FUNCTION_BLOCK PROCESS
VAR_INPUT
	ENABLE:BOOL;
	NEXTSTEP_EN:BOOL;
	Alarm_RST:BOOL;
	PMStableTime:INT;
	STEP_DATA:RecipeEachStep;
END_VAR
VAR_OUTPUT
	
	//APC
	APC_PRESSURE:REAL;
	APC_POSITION:REAL;
	APC_CONTROL_MODE:SINT;
	
	//MFC
	MFC1_SV:REAL;
	MFC2_SV:REAL;
	MFC3_SV:REAL;
	MFC4_SV:REAL;
	MFC5_SV:REAL;
	MFC6_SV:REAL;
	MFC7_SV:REAL;
	MFC8_SV:REAL;	
	MFC9_SV:REAL;	
	
	//HEATER
	WALL_TEMP:REAL;
	LID_TEMP:REAL;
	STAGE_TEMP1,
	STAGE_TEMP2,
	STAGE_TEMP3,
	STAGE_TEMP4:REAL;
	
	//STEP
	STEP_TIME_OUT:BOOL;
	STEP_ERR:BOOL;
	NEXTSTEP:BOOL;
	
	//Tolerance
	PRESSURE_WARNING:BOOL;
	PRESSURE_ALARM:BOOL;
	
	MFC1_WARNING:BOOL;
	MFC1_Alarm:BOOL;
	
	MFC2_WARNING:BOOL;
	MFC2_Alarm:BOOL;
	
	MFC3_WARNING:BOOL;
	MFC3_Alarm:BOOL;
	
	MFC4_WARNING:BOOL;
	MFC4_Alarm:BOOL;
	
	MFC5_WARNING:BOOL;
	MFC5_Alarm:BOOL;
	
	MFC6_WARNING:BOOL;
	MFC6_Alarm:BOOL;
	
	MFC7_WARNING:BOOL;
	MFC7_Alarm:BOOL;
	
	MFC8_WARNING:BOOL;
	MFC8_Alarm:BOOL;
	
	MFC9_WARNING:BOOL;
	MFC9_Alarm:BOOL;
	
	WALL_TEMP_WARNING:BOOL;
	WALL_TEMP_Alarm:BOOL;
		
	LID_TEMP_WARNING:BOOL;
	LID_TEMP_Alarm:BOOL;
	
	STAGE_TEMP1_WARNING:BOOL;
	STAGE_TEMP1_Alarm:BOOL;
	
	STAGE_TEMP2_WARNING:BOOL;
	STAGE_TEMP2_Alarm:BOOL;
	
	STAGE_TEMP3_WARNING:BOOL;
	STAGE_TEMP3_Alarm:BOOL;
	
	STAGE_TEMP4_WARNING:BOOL;
	STAGE_TEMP4_Alarm:BOOL;
	
END_VAR
VAR
	STEP_TIME:TON;
	STEP_TIME_DONE:BOOL;
	
	COMPLETION:INT;
	
	//Tolerance
	TOL_PRESSURE_PERCENT:Tolerance;
	TOL_PRESSURE_VALUE_EN:BOOL;
	TOL_PRESSURE_PERCENT_EN:BOOL;
	
	TOL_MFC1:Tolerance;
	TOL_MFC2:Tolerance;
	TOL_MFC3:Tolerance;
	//TOL_MFC4:Tolerance;
	TOL_MFC5:Tolerance;
	TOL_MFC6:Tolerance;
	TOL_MFC7:Tolerance;
	//TOL_MFC8:Tolerance;
	//TOL_MFC9:Tolerance;
	TOL_MFC_VALUE_EN:BOOL;
	TOL_MFC_PERCENT_EN:BOOL;

	TOL_WALL_TEMP:Tolerance;

	TOL_LID_TEMP:Tolerance;

	TOL_STAGE_TEMP1:Tolerance;	
	TOL_STAGE_TEMP2:Tolerance;
	TOL_STAGE_TEMP3:Tolerance;	
	TOL_STAGE_TEMP4:Tolerance;
	
	TOL_HEATER_VALUE_EN:BOOL;
	TOL_HEATER_PERCENT_EN:BOOL;
	
	TON_STEP_TIME:TON;
	TON_STEP_TIME_EN:BOOL;
	
	WARNING_OCC:BOOL;
	ALARM_OCC:BOOL;
	
	i:INT;
	
	STABLE_DONE:BOOL;
	EN_TRIG:R_TRIG;
	TON_STABLE_PROCESS:TON;
	
	CHAMBER_TEMP_MIN_VALUE:REAL;
	STAGE_EDGE_TEMP_MIN_VALUE:REAL;
	STAGE_CENTER_TEMP_MIN_VALUE:REAL;
		
END_VAR

//NOT ENABLE
	IF NOT ENABLE 
		THEN
		i:=0;
		STEP_ERR:=FALSE;
		STEP_TIME_OUT:=FALSE;
		NEXTSTEP:=FALSE;
		TON_STEP_TIME_EN:=FALSE;
	END_IF;
	
//初始化
	EN_TRIG(CLK:= ENABLE, Q=> );
	IF EN_TRIG.Q OR NEXTSTEP_EN
		THEN
		i:=1;
		STEP_ERR:=FALSE;
		STEP_TIME_OUT:=FALSE;
		NEXTSTEP:=FALSE;
		TON_STEP_TIME_EN:=TRUE;
	END_IF;

	
//STEP开始时赋值
	IF  ENABLE AND NOT STEP_TIME_DONE
	THEN
	//APC
	IF 		STEP_DATA.LstUnit.Pressure.PressureUnitMode = 'Pressure' 
			THEN
			APC_PRESSURE:=STEP_DATA.LstUnit.Pressure.StartValue;
			APC_CONTROL_MODE:=5;
			ELSIF 	
			STEP_DATA.LstUnit.Pressure.PressureUnitMode = 'Position'	
			THEN
			APC_POSITION:=STEP_DATA.LstUnit.Pressure.StartValue;
			APC_CONTROL_MODE:=2;
	END_IF
	
	IF 		STEP_DATA.LstUnit.Pressure.ToleranceMode = 'Value' 
			THEN
			TOL_PRESSURE_VALUE_EN:=TRUE;
			TOL_PRESSURE_PERCENT_EN:=FALSE;
			ELSIF 	
			STEP_DATA.LstUnit.Pressure.ToleranceMode = 'Percent'	
			THEN
			TOL_PRESSURE_VALUE_EN:=FALSE;
			TOL_PRESSURE_PERCENT_EN:=TRUE;
	END_IF
	
	//MFC
	IF 		STEP_DATA.LstUnit.GAS.ToleranceMode = 'Value' 
			THEN
			TOL_MFC_VALUE_EN:=TRUE;
			TOL_MFC_PERCENT_EN:=FALSE;
			ELSIF 	
			STEP_DATA.LstUnit.GAS.ToleranceMode = 'Percent'	
			THEN
			TOL_MFC_VALUE_EN:=FALSE;
			TOL_MFC_PERCENT_EN:=TRUE;
	END_IF
	
	MFC1_SV:=INT_TO_REAL(STEP_DATA.LstUnit.GAS.Gas1);
	MFC2_SV:=INT_TO_REAL(STEP_DATA.LstUnit.GAS.Gas2);
	MFC3_SV:=INT_TO_REAL(STEP_DATA.LstUnit.GAS.Gas3);
	MFC4_SV:=INT_TO_REAL(STEP_DATA.LstUnit.GAS.Gas4);	
	MFC5_SV:=INT_TO_REAL(STEP_DATA.LstUnit.GAS.Gas5);
	MFC6_SV:=INT_TO_REAL(STEP_DATA.LstUnit.GAS.Gas6);
	MFC7_SV:=INT_TO_REAL(STEP_DATA.LstUnit.GAS.Gas7);
	MFC8_SV:=INT_TO_REAL(STEP_DATA.LstUnit.GAS.Gas8);	
	MFC9_SV:=INT_TO_REAL(STEP_DATA.LstUnit.GAS.Gas9);
	
	//HEATER
	IF 		STEP_DATA.LstUnit.Heater.ToleranceMode = 'Value' 
			THEN
			TOL_HEATER_VALUE_EN:=TRUE;
			TOL_HEATER_PERCENT_EN:=FALSE;
			ELSIF 	
			STEP_DATA.LstUnit.Heater.ToleranceMode = 'Percent'	
			THEN
			TOL_HEATER_VALUE_EN:=FALSE;
			TOL_HEATER_PERCENT_EN:=TRUE;
	END_IF
	
	WALL_TEMP:=INT_TO_REAL(STEP_DATA.LstUnit.Heater.WallTemp);
	LID_TEMP:=INT_TO_REAL(STEP_DATA.LstUnit.Heater.LidTemp);
	STAGE_TEMP1:=INT_TO_REAL(STEP_DATA.LstUnit.Heater.StageTemp1);
	STAGE_TEMP2:=INT_TO_REAL(STEP_DATA.LstUnit.Heater.StageTemp2);
	STAGE_TEMP3:=INT_TO_REAL(STEP_DATA.LstUnit.Heater.StageTemp3);
	STAGE_TEMP4:=INT_TO_REAL(STEP_DATA.LstUnit.Heater.StageTemp4);
	END_IF;
	
// Lifter
	GV.NDO.AV110 :=	STEP_DATA.Lifter_Up AND NOT STEP_DATA.Lifter_Down;
	GV.NDO.AV109 :=	FALSE;
	
//取最小值
		IF 
		GV.AI.Chamber_Temp1<=GV.AI.Chamber_Temp2 AND GV.AI.Chamber_Temp1<=GV.AI.Chamber_Temp3
		THEN 
		CHAMBER_TEMP_MIN_VALUE:=GV.AI.Chamber_Temp1;
		ELSIF 
		GV.AI.Chamber_Temp2<=GV.AI.Chamber_Temp1 AND GV.AI.Chamber_Temp2<=GV.AI.Chamber_Temp3
		THEN
		CHAMBER_TEMP_MIN_VALUE:=GV.AI.Chamber_Temp2;
		ELSIF
		GV.AI.Chamber_Temp3<=GV.AI.Chamber_Temp2 AND GV.AI.Chamber_Temp3<=GV.AI.Chamber_Temp1
		THEN
		CHAMBER_TEMP_MIN_VALUE:=GV.AI.Chamber_Temp3;
	END_IF
	
//Tolerance
	TOL_PRESSURE_PERCENT(
		ENABLE:= TOL_PRESSURE_PERCENT.SV>0	AND ENABLE,
		STEP_TYPE:=	STEP_DATA.Completion,
		STEP_TIME:=	STEP_DATA.StepTime+STEP_DATA.AddTime,
		TOL_V:= TOL_PRESSURE_VALUE_EN, 
		TOL_P:= TOL_PRESSURE_PERCENT_EN, 
		SV:= STEP_DATA.LstUnit.Pressure.StartValue, 
		PV:= GV.AI.	APC.ACTUAL_PRESSURE, 
		WARNING_RANGE:= STEP_DATA.LstUnit.Pressure.StartValueWarningRange, 
		ALARM_RANGE:= STEP_DATA.LstUnit.Pressure.StartValueAlarmRange, 
		DELAY_TIME:=STEP_DATA.LstUnit.Pressure.ToleranceDelayTime,
		RST	:=	Alarm_RST,
		STABLE_TIME := PMStableTime,
		STU_WARNING=> PRESSURE_WARNING, 
		STU_ALARM=> PRESSURE_ALARM, );

	TOL_MFC1(
		ENABLE:= TOL_MFC1.SV>0	AND ENABLE,
		STEP_TYPE:=	STEP_DATA.Completion,
		STEP_TIME:=	STEP_DATA.StepTime+STEP_DATA.AddTime,
		TOL_V:= TOL_MFC_VALUE_EN, 
		TOL_P:= TOL_MFC_PERCENT_EN, 
		SV:= STEP_DATA.LstUnit.GAS.Gas1, 
		PV:= GV.AI.MFC1_Flow, 
		WARNING_RANGE:= STEP_DATA.LstUnit.GAS.Gas1WarningRange, 
		ALARM_RANGE:= STEP_DATA.LstUnit.GAS.Gas1AlarmRange, 
		DELAY_TIME:=STEP_DATA.LstUnit.GAS.ToleranceDelayTime,
		RST	:=	Alarm_RST,
		STABLE_TIME := PMStableTime,
		STU_WARNING=> MFC1_WARNING, 
		STU_ALARM=> MFC1_Alarm, );
(*	
	TOL_MFC2(
		ENABLE:= TOL_MFC2.SV>0	AND ENABLE,
		STEP_TYPE:=	STEP_DATA.Completion,
		STEP_TIME:=	STEP_DATA.StepTime+STEP_DATA.AddTime,
		TOL_V:= TOL_MFC_VALUE_EN, 
		TOL_P:= TOL_MFC_PERCENT_EN, 
		SV:= STEP_DATA.LstUnit.GAS.Gas2, 
		PV:= GV.AI.MFC2_Flow,
		WARNING_RANGE:= STEP_DATA.LstUnit.GAS.Gas2WarningRange, 
		ALARM_RANGE:= STEP_DATA.LstUnit.GAS.Gas2AlarmRange,  
		DELAY_TIME:=STEP_DATA.LstUnit.GAS.ToleranceDelayTime,
		RST	:=	Alarm_RST,
		STABLE_TIME := PMStableTime,
		STU_WARNING=> MFC2_WARNING, 
		STU_ALARM=> MFC2_Alarm, );
	
	TOL_MFC3(
		ENABLE:= TOL_MFC3.SV>0	AND ENABLE,
		STEP_TYPE:=	STEP_DATA.Completion,
		STEP_TIME:=	STEP_DATA.StepTime+STEP_DATA.AddTime,
		TOL_V:= TOL_MFC_VALUE_EN, 
		TOL_P:= TOL_MFC_PERCENT_EN, 
		SV:= STEP_DATA.LstUnit.GAS.Gas3, 
		PV:= GV.AI.MFC3_Flow,
		WARNING_RANGE:= STEP_DATA.LstUnit.GAS.Gas3WarningRange, 
		ALARM_RANGE:= STEP_DATA.LstUnit.GAS.Gas3AlarmRange, 
		DELAY_TIME:=STEP_DATA.LstUnit.GAS.ToleranceDelayTime,
		RST	:=	Alarm_RST,
		STABLE_TIME := PMStableTime,
		STU_WARNING=> MFC3_WARNING, 
		STU_ALARM=> MFC3_Alarm, );
	
	
	TOL_MFC5(
		ENABLE:= TOL_MFC5.SV>0	AND ENABLE,
		STEP_TYPE:=	STEP_DATA.Completion,
		STEP_TIME:=	STEP_DATA.StepTime+STEP_DATA.AddTime,
		TOL_V:= TOL_MFC_VALUE_EN, 
		TOL_P:= TOL_MFC_PERCENT_EN, 
		SV:= STEP_DATA.LstUnit.GAS.Gas5, 
		PV:= GV.AI.MFC5_Flow,
		WARNING_RANGE:= STEP_DATA.LstUnit.GAS.Gas5WarningRange, 
		ALARM_RANGE:= STEP_DATA.LstUnit.GAS.Gas5AlarmRange, 
		DELAY_TIME:=STEP_DATA.LstUnit.GAS.ToleranceDelayTime,
		RST	:=	Alarm_RST, 
		STABLE_TIME := PMStableTime,
		STU_WARNING=> MFC5_WARNING, 
		STU_ALARM=> MFC5_Alarm, );
	
	TOL_MFC6(
		ENABLE:= TOL_MFC6.SV>0	AND ENABLE,
		STEP_TYPE:=	STEP_DATA.Completion,
		STEP_TIME:=	STEP_DATA.StepTime+STEP_DATA.AddTime,
		TOL_V:= TOL_MFC_VALUE_EN, 
		TOL_P:= TOL_MFC_PERCENT_EN, 
		SV:= STEP_DATA.LstUnit.GAS.Gas6, 
		PV:= GV.AI.MFC6_Flow,
		WARNING_RANGE:= STEP_DATA.LstUnit.GAS.Gas6WarningRange, 
		ALARM_RANGE:= STEP_DATA.LstUnit.GAS.Gas6AlarmRange, 
		DELAY_TIME:=STEP_DATA.LstUnit.GAS.ToleranceDelayTime,
		RST	:=	Alarm_RST,
		STABLE_TIME := PMStableTime,
		STU_WARNING=> MFC6_WARNING, 
		STU_ALARM=> MFC6_Alarm, );
	
	TOL_MFC7(
		ENABLE:= TOL_MFC7.SV>0	AND ENABLE,
		STEP_TYPE:=	STEP_DATA.Completion,
		STEP_TIME:=	STEP_DATA.StepTime+STEP_DATA.AddTime,
		TOL_V:= TOL_MFC_VALUE_EN, 
		TOL_P:= TOL_MFC_PERCENT_EN, 
		SV:= STEP_DATA.LstUnit.GAS.Gas7, 
		PV:= GV.AI.MFC7_Flow,
		WARNING_RANGE:= STEP_DATA.LstUnit.GAS.Gas7WarningRange, 
		ALARM_RANGE:= STEP_DATA.LstUnit.GAS.Gas7AlarmRange, 
		DELAY_TIME:=STEP_DATA.LstUnit.GAS.ToleranceDelayTime,
		RST	:=	Alarm_RST,
		STABLE_TIME := PMStableTime,
		STU_WARNING=> MFC7_WARNING, 
		STU_ALARM=> MFC7_Alarm, );
*)
	TOL_WALL_TEMP(
		ENABLE:= ENABLE,
		STEP_TYPE:=	STEP_DATA.Completion,
		STEP_TIME:=	STEP_DATA.StepTime+STEP_DATA.AddTime,
		TOL_V:= TOL_HEATER_VALUE_EN, 
		TOL_P:= TOL_HEATER_PERCENT_EN, 
		SV:= STEP_DATA.LstUnit.Heater.WallTemp, 
		PV:= CHAMBER_TEMP_MIN_VALUE, 
		WARNING_RANGE:= STEP_DATA.LstUnit.Heater.WallTempWaningRange, 
		ALARM_RANGE:= STEP_DATA.LstUnit.Heater.WallTempAlarmRange, 
		DELAY_TIME:=STEP_DATA.LstUnit.Heater.ToleranceDelayTime,
		RST	:=	Alarm_RST,
		STABLE_TIME := PMStableTime,
		STU_WARNING=> WALL_TEMP_WARNING, 
		STU_ALARM=> WALL_TEMP_Alarm, );
	
	TOL_LID_TEMP(
		ENABLE:= ENABLE,
		STEP_TYPE:=	STEP_DATA.Completion,
		STEP_TIME:=	STEP_DATA.StepTime+STEP_DATA.AddTime,
		TOL_V:= TOL_HEATER_VALUE_EN, 
		TOL_P:= TOL_HEATER_PERCENT_EN,
		SV:= STEP_DATA.LstUnit.Heater.LidTemp, 
		PV:= GV.AI.	Lid_Temp, 
		WARNING_RANGE:= STEP_DATA.LstUnit.Heater.LidTempWaningRange, 
		ALARM_RANGE:= STEP_DATA.LstUnit.Heater.LidTempAlarmRange, 
		DELAY_TIME:=STEP_DATA.LstUnit.Heater.ToleranceDelayTime,
		RST	:=	Alarm_RST,
		STABLE_TIME := PMStableTime,
		STU_WARNING=> LID_TEMP_WARNING, 
		STU_ALARM=> LID_TEMP_Alarm, );
		
	
	TOL_STAGE_TEMP1(
		ENABLE:= ENABLE,
		STEP_TYPE:=	STEP_DATA.Completion,
		STEP_TIME:=	STEP_DATA.StepTime+STEP_DATA.AddTime,
		TOL_V:= TOL_HEATER_VALUE_EN, 
		TOL_P:= TOL_HEATER_PERCENT_EN,
		SV:= STEP_DATA.LstUnit.Heater.StageTemp1, 
		PV:= GV.AI.Stage_Temp1, 
		WARNING_RANGE:= STEP_DATA.LstUnit.Heater.StageTemp1WaningRange, 
		ALARM_RANGE:= STEP_DATA.LstUnit.Heater.StageTemp1AlarmRange, 
		DELAY_TIME:=STEP_DATA.LstUnit.Heater.ToleranceDelayTime,
		RST	:=	Alarm_RST,
		STABLE_TIME := PMStableTime,
		STU_WARNING=> STAGE_TEMP1_WARNING, 
		STU_ALARM=> STAGE_TEMP1_Alarm, );
	
	TOL_STAGE_TEMP2(
		ENABLE:= ENABLE,
		STEP_TYPE:=	STEP_DATA.Completion,
		STEP_TIME:=	STEP_DATA.StepTime+STEP_DATA.AddTime,
		TOL_V:= TOL_HEATER_VALUE_EN, 
		TOL_P:= TOL_HEATER_PERCENT_EN,
		SV:= STEP_DATA.LstUnit.Heater.StageTemp2, 
		PV:= GV.AI.Stage_Temp2, 
		WARNING_RANGE:= STEP_DATA.LstUnit.Heater.StageTemp2WaningRange, 
		ALARM_RANGE:= STEP_DATA.LstUnit.Heater.StageTemp2AlarmRange,
		DELAY_TIME:=STEP_DATA.LstUnit.Heater.ToleranceDelayTime,
		RST	:=	Alarm_RST, 
		STABLE_TIME := PMStableTime,
		STU_WARNING=> STAGE_TEMP2_WARNING, 
		STU_ALARM=> STAGE_TEMP2_Alarm, );
		
	TOL_STAGE_TEMP3(
		ENABLE:= ENABLE,
		STEP_TYPE:=	STEP_DATA.Completion,
		STEP_TIME:=	STEP_DATA.StepTime+STEP_DATA.AddTime,
		TOL_V:= TOL_HEATER_VALUE_EN, 
		TOL_P:= TOL_HEATER_PERCENT_EN,
		SV:= STEP_DATA.LstUnit.Heater.StageTEMP3, 
		PV:= GV.AI.Stage_TEMP3, 
		WARNING_RANGE:= STEP_DATA.LstUnit.Heater.StageTEMP3WaningRange, 
		ALARM_RANGE:= STEP_DATA.LstUnit.Heater.StageTEMP3AlarmRange, 
		DELAY_TIME:=STEP_DATA.LstUnit.Heater.ToleranceDelayTime,
		RST	:=	Alarm_RST,
		STABLE_TIME := PMStableTime,
		STU_WARNING=> STAGE_TEMP3_WARNING, 
		STU_ALARM=> STAGE_TEMP3_Alarm, );
	
	TOL_STAGE_TEMP4(
		ENABLE:= ENABLE,
		STEP_TYPE:=	STEP_DATA.Completion,
		STEP_TIME:=	STEP_DATA.StepTime+STEP_DATA.AddTime,
		TOL_V:= TOL_HEATER_VALUE_EN, 
		TOL_P:= TOL_HEATER_PERCENT_EN,
		SV:= STEP_DATA.LstUnit.Heater.StageTEMP4, 
		PV:= GV.AI.Stage_TEMP4, 
		WARNING_RANGE:= STEP_DATA.LstUnit.Heater.StageTEMP4WaningRange, 
		ALARM_RANGE:= STEP_DATA.LstUnit.Heater.StageTEMP4AlarmRange,
		DELAY_TIME:=STEP_DATA.LstUnit.Heater.ToleranceDelayTime,
		RST	:=	Alarm_RST, 
		STABLE_TIME := PMStableTime,
		STU_WARNING=> STAGE_TEMP4_WARNING, 
		STU_ALARM=> STAGE_TEMP4_Alarm, );


		
		
		
//ALRAM & WARNING	
	WARNING_OCC:=  PRESSURE_WARNING 
				OR MFC1_WARNING OR MFC2_WARNING OR MFC3_WARNING OR MFC4_WARNING OR MFC5_WARNING
				OR MFC6_WARNING OR MFC7_WARNING OR MFC8_WARNING OR MFC9_WARNING 
				OR WALL_TEMP_WARNING OR LID_TEMP_WARNING OR STAGE_TEMP1_WARNING 
				OR STAGE_TEMP1_WARNING OR STAGE_TEMP2_WARNING OR STAGE_TEMP3_WARNING OR STAGE_TEMP4_WARNING;
	
	ALARM_OCC:=    PRESSURE_ALARM 				
				OR MFC1_ALARM OR MFC2_ALARM OR MFC3_ALARM OR MFC4_ALARM OR MFC5_ALARM
				OR MFC6_ALARM OR MFC7_ALARM OR MFC8_ALARM OR MFC9_ALARM 
				OR WALL_TEMP_ALARM OR LID_TEMP_ALARM OR STAGE_TEMP1_Alarm 
				OR STAGE_TEMP1_ALARM OR STAGE_TEMP2_ALARM OR STAGE_TEMP3_ALARM OR STAGE_TEMP4_ALARM;

//STABLE DONE
TON_STABLE_PROCESS(IN:= ENABLE, PT:= INT_TO_TIME(PMStableTime)*1000, Q=> , ET=> );

	STABLE_DONE:=	TOL_PRESSURE_PERCENT.STABLE_DONE 
				AND TOL_MFC1.STABLE_DONE 
				AND TOL_MFC2.STABLE_DONE 
				AND TOL_MFC3.STABLE_DONE 
				AND TOL_MFC5.STABLE_DONE 			 
				AND TOL_MFC6.STABLE_DONE 
				AND TOL_MFC7.STABLE_DONE
				AND TOL_WALL_TEMP.STABLE_DONE
				AND TOL_LID_TEMP.STABLE_DONE
				AND TOL_STAGE_TEMP1.STABLE_DONE
				AND TOL_STAGE_TEMP2.STABLE_DONE
				AND TOL_STAGE_TEMP3.STABLE_DONE
				AND TOL_STAGE_TEMP4.STABLE_DONE
				AND TON_STABLE_PROCESS.Q;

//STEP流程	
	CASE i OF
	1:	IF STEP_DATA.Completion='Stable'
			THEN
			i:= 10;
			ELSIF STEP_DATA.Completion='Time'
			THEN
			i:= 20;
		END_IF
	
		//STABLE
	10:	IF 	STABLE_DONE 
			THEN i:=100; 
		END_IF;
			
		//TIME
	20:	IF 	ALARM_OCC 
			THEN i:=50; 
			ELSE i:=21;
		END_IF;	
		
	21:	IF 	STEP_TIME_DONE 
			THEN i:= 100;		
			ELSE i:= 20;	
		END_IF;
		
		//ALARM CONDITION
	50:	STEP_ERR:=TRUE;
		TON_STEP_TIME_EN:=FALSE;
	
		//TIME OUT
	51: STEP_TIME_OUT:=TRUE;
		TON_STEP_TIME_EN:=FALSE;
		
		//FINISHED
	100:	NEXTSTEP:=TRUE;
		TON_STEP_TIME_EN:=FALSE;	
	END_CASE;	
	
//PROCESS TIME
	STEP_TIME(IN:= TON_STEP_TIME_EN, PT:= INT_TO_TIME(STEP_DATA.StepTime+STEP_DATA.AddTime)*1000, Q=> STEP_TIME_DONE, ET=> );

END_FUNCTION_BLOCK
